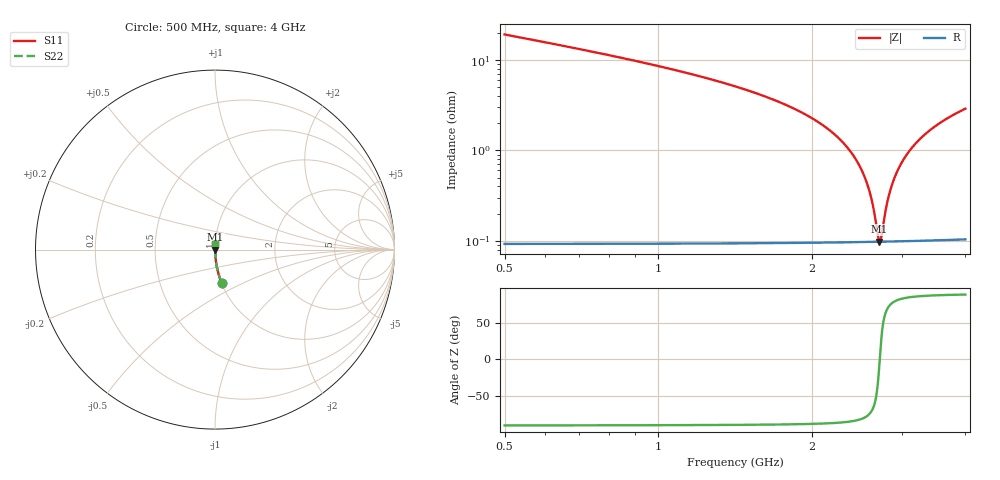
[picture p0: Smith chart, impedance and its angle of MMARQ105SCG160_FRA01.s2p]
! MMARQ105SCG160_FRA01  S-PARAMETER MODEL  ( General Type )
! Model Generated by TAIYO YUDEN Corporation (http://www.ty-top.com)
! Version 1.0
! TAIYO YUDEN Control No. 200326
! Copyright(c) 2020 TAIYO YUDEN CO.,LTD. All Rights Reserved.
! Product Description (link to TY-COMPAS)
! https://ds.yuden.co.jp/TYCOMPAS/or/detail?pn=MMARQ105SCG160JFRA01&u=M
! Products Name : Multilayer Ceramic Capacitors
! Characteristics :
!  Capacitance : 16 pF , Rated Voltage : 250V , TCC : CG / C0G
!  Case Size : 1.0 x 0.5 / 0.039 x 0.02 [mm/inch] , Thickness : 0.5 / 0.02 [mm/inch]
!  (Conditions: Temperature = 25 degC , DC Bias Current/Voltage = 0A / 0V)
! External Node Assignments :
!  1  o---| |---o  2
! GND o---------o GND
! Frequency Range : 500MHz  -  4GHz  [ 401 STEP ]
# MHz S RI R 50
! Freq[MHz].  S11 Real  S11 Imag  S21 Real  S21 Imag  S12 Real  S12 Imag  S22 Real  S22 Imag
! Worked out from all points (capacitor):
!   401 points, 500 MHz to 4 GHz, reference 50 ohm
!   read as one part in series: C = 16 pF near 517.5 MHz
!   lowest |Z| = 98.1 mohm at 2.714 GHz (marker M1)
!   series resonance near 2.718 GHz, so ESL is about 210 pH
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500  0.0364 -0.185  0.9636 0.185  0.9636 0.185  0.0364 -0.185
762.5  0.0151 -0.1182  0.9849 0.1182  0.9849 0.1182  0.0151 -0.1182
1086.25  0.00679 -0.0763  0.9932 0.0763  0.9932 0.0763  0.00679 -0.0763
1672.5  0.0023 -0.0368  0.9977 0.0368  0.9977 0.0368  0.0023 -0.0368
2005  0.00146 -0.0225  0.9985 0.0225  0.9985 0.0225  0.00146 -0.0225
2250  0.00115 -0.0139  0.9988 0.0139  0.9988 0.0139  0.00115 -0.0139
2416.25  0.00104 -0.0086  0.999 0.0086  0.999 0.0086  0.00104 -0.0086
2538.75  0.000993 -0.00498  0.999 0.00498  0.999 0.00498  0.000993 -0.00498
2617.5  0.000978 -0.00274  0.999 0.00274  0.999 0.00274  0.000978 -0.00274
2652.5  0.000975 -0.00177  0.999 0.00177  0.999 0.00177  0.000975 -0.00177
2696.25  0.000974 -0.000577  0.999 0.000577  0.999 0.000577  0.000974 -0.000577
2713.75  0.000974 -0.000105  0.999 0.000105  0.999 0.000105  0.000974 -0.000105
2722.5  0.000975 0.00013  0.999 -0.00013  0.999 -0.00013  0.000975 0.00013
2740  0.000976 0.000598  0.999 -0.000598  0.999 -0.000598  0.000976 0.000598
2792.5  0.000982 0.00198  0.999 -0.00198  0.999 -0.00198  0.000982 0.00198
2836.25  0.000989 0.00312  0.999 -0.00312  0.999 -0.00312  0.000989 0.00312
2923.75  0.00101 0.00534  0.999 -0.00534  0.999 -0.00534  0.00101 0.00534
3046.25  0.00106 0.00835  0.9989 -0.00835  0.9989 -0.00835  0.00106 0.00835
3212.5  0.00115 0.0123  0.9989 -0.0123  0.9989 -0.0123  0.00115 0.0123
3422.5  0.00129 0.017  0.9987 -0.017  0.9987 -0.017  0.00129 0.017
3685  0.00153 0.0226  0.9985 -0.0226  0.9985 -0.0226  0.00153 0.0226
4000  0.00187 0.0289  0.9981 -0.0289  0.9981 -0.0289  0.00187 0.0289
